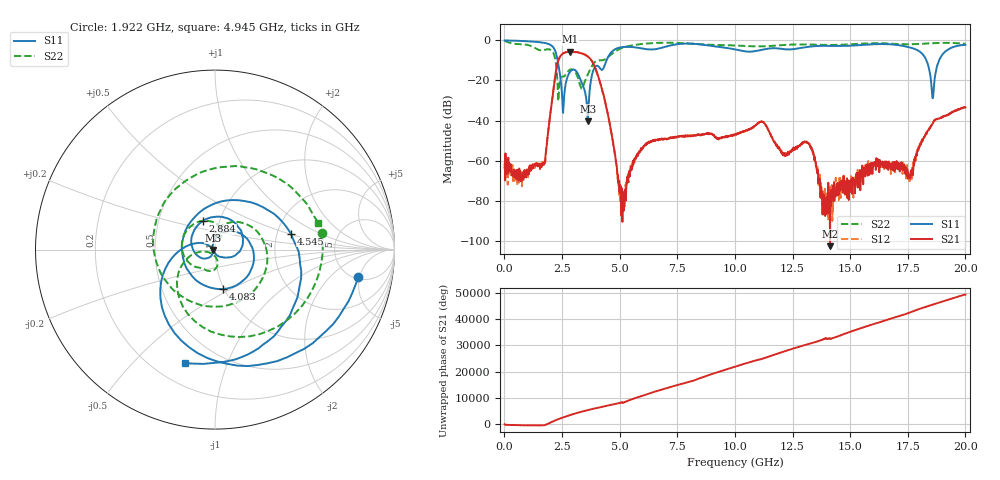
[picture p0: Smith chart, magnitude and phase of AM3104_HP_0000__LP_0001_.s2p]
!Created with skrf (http://scikit-rf.org).
# Hz S RI R 50.0
!freq ReS11 ImS11 ReS21 ImS21 ReS12 ImS12 ReS22 ImS22
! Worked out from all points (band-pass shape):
!   1601 points, 10 MHz to 20 GHz, reference 50 ohm
!   highest |S21| = -5.67 dB at 2.846 GHz (marker M1); lowest = -102.8 dB at 14.13 GHz (marker M2)
!   |S21| within 3 dB of the highest: 2.385 GHz to 3.689 GHz (1.304 GHz wide, 42.9 % of centre)
!   lowest |S11| = -40.3 dB at 3.621 GHz (marker M3), VSWR 1.02, Z = 49.1 - j0.231 ohm
!   |S11| at or under -10 dB: 2.311 GHz to 4.431 GHz (2.119 GHz wide, 62.9 % of centre); 18.31 GHz to 18.86 GHz (549.5 MHz wide, 2.96 % of centre)
!   |S22| runs from -30.3 to -0.2 dB; largest |S21 - S12| = 0.0044
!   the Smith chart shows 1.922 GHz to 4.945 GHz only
!   S11 on the Smith chart (normalised r, x): 1.922 GHz: 5.30, -4.81; 2.884 GHz: 0.83, +0.27; 4.083 GHz: 0.99, -0.46; 4.545 GHz: 2.38, +0.52; 4.945 GHz: 0.32, -0.71
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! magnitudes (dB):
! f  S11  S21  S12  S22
! 10 MHz  0.0  -63.4  -64.4  -0.2
! 1.647 GHz  -1.1  -61.4  -61.9  -4.9
! 1.922 GHz  -1.8  -43.5  -43.6  -4.4
! 2.546 GHz  -36.2  -6.5  -6.5  -18.1
! 2.846 GHz  -15.8  -5.7  -5.7  -14.6
! 2.884 GHz  -15.2  -5.7  -5.7  -14.5
! 3.346 GHz  -20.9  -6.4  -6.4  -24.0
! 3.621 GHz  -40.3  -8.0  -8.0  -16.9
! 4.083 GHz  -13.0  -18.4  -18.4  -10.0
! 4.545 GHz  -7.3  -40.1  -40.2  -7.9
! 4.945 GHz  -3.7  -71.0  -68.8  -4.5
! 5.17 GHz  -3.3  -76.0  -84.5  -3.5
! 6.682 GHz  -4.1  -49.5  -49.9  -1.2
! 10.01 GHz  -4.5  -47.0  -46.9  -2.5
! 13.34 GHz  -2.9  -54.3  -54.8  -2.1
! 13.79 GHz  -2.7  -76.0  -81.0  -2.2
! 14.13 GHz  -2.7  -102.8  -76.3  -2.2
! 16.68 GHz  -1.9  -60.5  -62.7  -1.5
! 17.61 GHz  -3.6  -68.5  -68.1  -1.9
! 18.59 GHz  -28.9  -41.5  -41.1  -1.4
! 19.03 GHz  -6.7  -38.0  -38.1  -1.2
! 20 GHz  -2.2  -33.4  -33.1  -1.6
